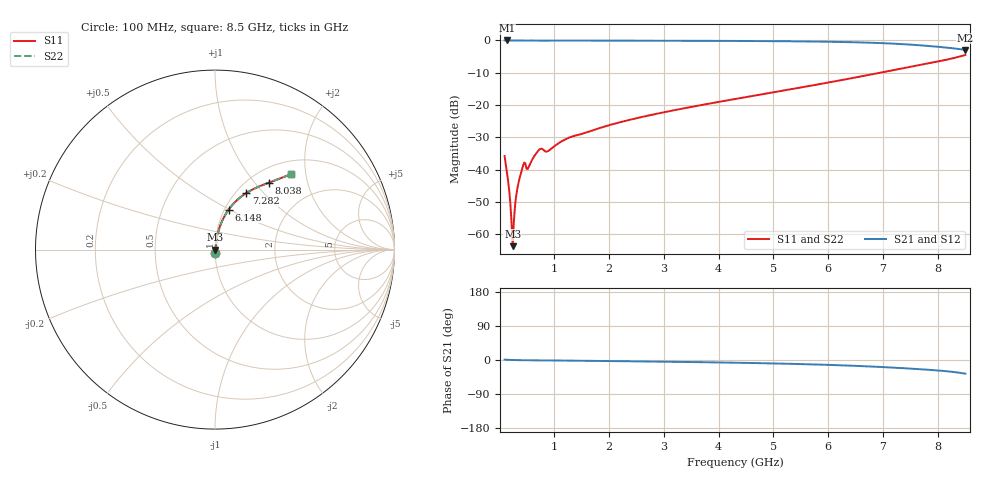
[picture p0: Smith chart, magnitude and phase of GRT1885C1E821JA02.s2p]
!Murata Part Number: GRT1885C1E821JA02
!These Parameters are Measured in Series Mode Connection
!Data Generated on Jun 19, 2026
!  o--ll--o
!Port1  Port2
!  o------o
!Operation Temp=25[degC], DC Bias Voltage=0[V]
!Freq. Start=100[MHz] Stop=9[GHz] 401[Steps]
# Hz S RI R 50
!Freq.(Hz) S11(Real) S11(Imag) S21(Real) S21(Imag) S12(Real) S12(Imag) S22(Real) S22(Imag)
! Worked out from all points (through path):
!   401 points, 100 MHz to 8.5 GHz, reference 50 ohm
!   highest |S21| = 0.00 dB at 142 MHz (marker M1); lowest = -2.9 dB at 8.5 GHz (marker M2)
!   group delay of S21, straight-line fit = 9.45 ps
!   lowest |S11| = -63.6 dB at 247 MHz (marker M3), VSWR 1.00, Z = 50.1 + j0.00327 ohm
!   |S11| at or under -10 dB: start of sweep to 6.943 GHz
!   |S22| runs from -63.6 to -4.5 dB; largest |S21 - S12| = 0
!   S11 on the Smith chart (normalised r, x): 100 MHz: 1.00, -0.03; 6.148 GHz: 1.05, +0.49; 7.282 GHz: 1.11, +0.81; 8.038 GHz: 1.23, +1.19; 8.5 GHz: 1.27, +1.65
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1e8  0.000661 -0.0162  0.9993 0.0162  0.9993 0.0162  0.000661 -0.0162
1.42e8  0.000531 -0.00918  0.9995 0.00918  0.9995 0.00918  0.000531 -0.00918
1.84e8  0.000536 -0.00471  0.9995 0.00471  0.9995 0.00471  0.000536 -0.00471
2.05e8  0.000564 -0.00296  0.9994 0.00296  0.9994 0.00296  0.000564 -0.00296
2.47e8  0.000656 3.27e-05  0.9993 -3.27e-05  0.9993 -3.27e-05  0.000656 3.27e-05
2.89e8  0.000794 0.0026  0.9992 -0.0026  0.9992 -0.0026  0.000794 0.0026
3.1e8  0.000885 0.00379  0.9991 -0.00379  0.9991 -0.00379  0.000885 0.00379
3.52e8  0.00113 0.0061  0.9989 -0.0061  0.9989 -0.0061  0.00113 0.0061
4.36e8  0.00292 0.0111  0.9971 -0.0111  0.9971 -0.0111  0.00292 0.0111
5.41e8  0.00303 0.0108  0.997 -0.0108  0.997 -0.0108  0.00303 0.0108
7.3e8  0.00596 0.0195  0.994 -0.0195  0.994 -0.0195  0.00596 0.0195
8.98e8  0.00585 0.0187  0.9942 -0.0187  0.9942 -0.0187  0.00585 0.0187
1.213e9  0.00589 0.0291  0.9941 -0.0291  0.9941 -0.0291  0.00589 0.0291
1.507e9  0.00748 0.035  0.9925 -0.035  0.9925 -0.035  0.00748 0.035
2.914e9  0.0126 0.0736  0.9874 -0.0736  0.9874 -0.0736  0.0126 0.0736
4.3e9  0.0251 0.1216  0.9749 -0.1216  0.9749 -0.1216  0.0251 0.1216
5.707e9  0.0568 0.193  0.9432 -0.193  0.9432 -0.193  0.0568 0.193
6.148e9  0.076 0.2227  0.924 -0.2227  0.924 -0.2227  0.076 0.2227
7.114e9  0.1532 0.3007  0.8468 -0.3007  0.8468 -0.3007  0.1532 0.3007
7.282e9  0.174 0.3149  0.826 -0.3149  0.826 -0.3149  0.174 0.3149
8.038e9  0.3009 0.3733  0.6991 -0.3733  0.6991 -0.3733  0.3009 0.3733
8.5e9  0.4244 0.4197  0.5756 -0.4197  0.5756 -0.4197  0.4244 0.4197
